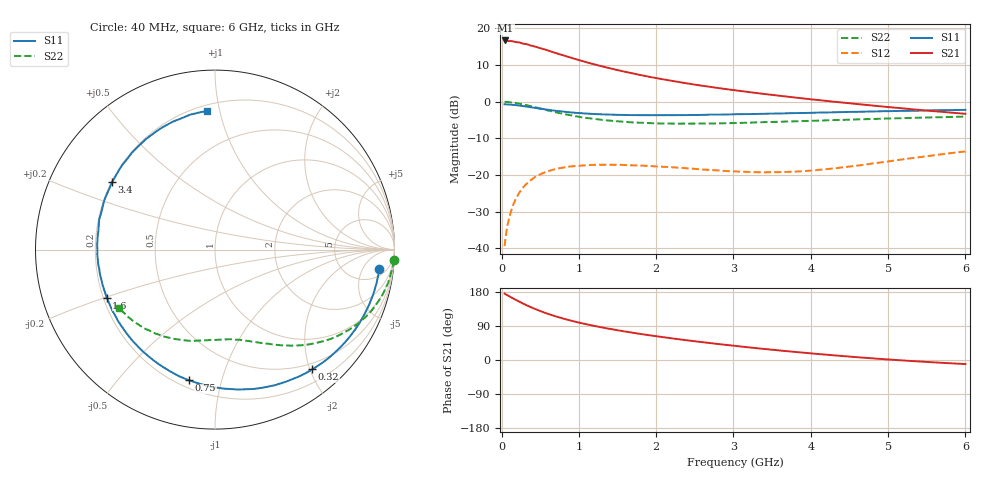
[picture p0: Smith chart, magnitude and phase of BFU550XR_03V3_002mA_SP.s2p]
! Filename:  P:\Prog\Test\Noise\ATS_data\Testdata_Net\03 Spar\BFU550XR_APG2013_45_C05_03p3V_002mA_SP_CM01_D.s2p
! Date/Time: Tue 06/Aug/2013 14:38:14
! BFU550XR_APG2013_45_C05_03p3V_1to35mA_SP_CM01_Bias2_R.s2p
! MDIF S-parameter v. bias file
! BFU550XR_APG2013_45_C05_03p3V_1to35mA_SP_CM01
! Date/time Fri Aug 02 14:41:13 2013
! VAR V_out= 3.3010
! VAR I_out= 2.0050
! VAR V_in= 0.7946
! VAR I_in= 0.0220
! Device data file deembeded for feedlines and parallel
! Original file: \03 Spar\BFU550XR_APG2013_45_C05_03p3V_002mA_SP_CM01_R.s2p
! Feed-files: PR006V01_02082013_Feed1.s2p, PR006V01_02082013_Feed2.s2p
! Parallel-file: PR006V01_02082013_Par.s2p
# MHz S MA R 50
!  Freq-MHz  S11-mag  S11-arg  S21-mag  S21-arg  S12-mag  S12-arg  S22-mag  S22-arg
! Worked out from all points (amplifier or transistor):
!   98 points, 40 MHz to 6 GHz, reference 50 ohm
!   highest |S21| = 16.7 dB at 50 MHz (marker M1)
!   |S21| within 3 dB of that: start of sweep to 637.4 MHz
!   unconditionally stable (mu >= 1): 3.049 GHz to 4.772 GHz
!   at 300 MHz: K = 0.10, MSG = 19.3 dB, |S12| = -22.9 dB
!   at 1.6 GHz: K = 0.50, MSG = 12.7 dB, |S12| = -17.3 dB
!   at 6 GHz: K = 0.83, MSG = 5.1 dB, |S12| = -13.6 dB
!   S11 on the Smith chart (normalised r, x): 40 MHz: 8, -12; 320 MHz: 0.40, -2.04; 750 MHz: 0.24, -0.79; 1.6 GHz: 0.21, -0.20; 3.4 GHz: 0.20, +0.29; 6 GHz: 0.24, +0.91
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40  0.9226 -6.7  6.841 175.6  0.0107 85.7  0.9963 -3.4
50  0.9211 -8.3  6.852 173.5  0.01332 84.7  0.9961 -4.5
90  0.9167 -14.9  6.717 169.2  0.02379 80.9  0.9878 -8.2
120  0.9117 -19.9  6.738 165.8  0.03146 78.0  0.9821 -11.0
220  0.8893 -35.9  6.461 155.0  0.05509 68.8  0.9452 -19.4
280  0.873 -44.7  6.192 148.8  0.06771 63.5  0.9192 -24.1
320  0.8595 -50.9  6.12 144.9  0.07522 60.3  0.8986 -27.1
440  0.8227 -67.2  5.633 134.2  0.09446 51.6  0.8384 -34.8
550  0.7898 -80.7  5.198 125.5  0.1075 44.7  0.7829 -41.0
650  0.7649 -91.5  4.798 118.5  0.1169 39.5  0.7406 -45.6
750  0.7423 -101.3  4.439 112.2  0.1238 35.0  0.701 -49.6
900  0.7143 -114.4  3.982 103.8  0.1311 29.2  0.6527 -54.9
1050  0.6952 -125.5  3.575 96.5  0.1348 24.4  0.611 -59.5
1300  0.6727 -141.0  3.041 86.0  0.138 18.2  0.5658 -65.8
1600  0.6598 -156.1  2.56 75.1  0.1369 12.9  0.5308 -72.4
2050  0.6556 -174.0  2.055 61.4  0.1301 8.6  0.5054 -81.1
2500  0.6579 171.1  1.712 49.4  0.1214 7.3  0.5031 -89.2
3100  0.6766 154.3  1.398 35.5  0.1112 12.0  0.5145 -99.7
3400  0.6854 146.8  1.275 29.1  0.1089 16.0  0.5269 -105.1
4100  0.7109 130.6  1.054 15.8  0.1176 27.6  0.5524 -117.1
5200  0.7508 108.0  0.81 -1.3  0.1643 36.2  0.5971 -135.7
6000  0.7744 93.4  0.6846 -10.7  0.2097 34.1  0.6264 -148.9
